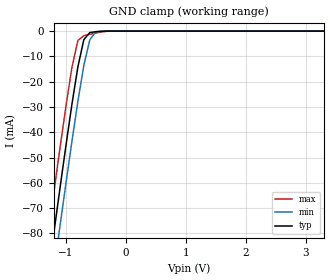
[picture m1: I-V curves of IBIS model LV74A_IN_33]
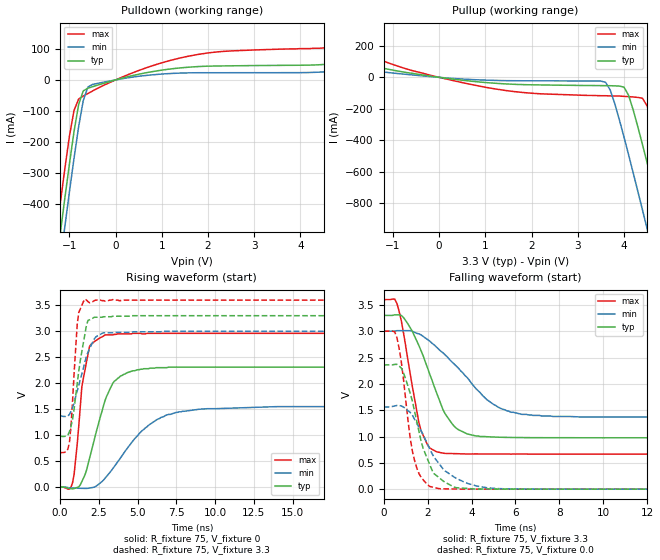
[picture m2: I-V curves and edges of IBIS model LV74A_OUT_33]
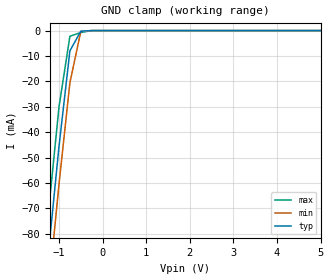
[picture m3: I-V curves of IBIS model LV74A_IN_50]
| TEXAS INSTRUMENTS INCORPORATED
| Standard Linear and Logic Group
| IBIS Model of SN74LV74A
| DUAL POSITIVE-EDGE-TRIGGERED D-TYPE FLIP-FLOPS
| SOIC 14-pin (D), SOP 14-pin (NS), SSOP 14-pin (DB), TSSOP 14-pin (PW)
| and TVSOP 14-pin (DGV) Package
[IBIS Ver]   3.2
[Comment Char]  |_char
[File Name]   sn74lv74a.ibs
[File Rev]   2.1 H_die
[Date]   Nov, 10 2004
[Source]   Data created from HSPICE simulations at TI-SLL.
[Notes]   The following is an IBIS list for the LV74A.
   - FILE REV HISTORY
   - 2.1 Re-Release IBIS file on 11/22/04
   - Power clamp data deleted as there is no power-clamp diode
|   Please contact sllibis@ti.com with questions and
|   comments concerning SLL IBIS models.
[Disclaimer] Property of Texas Instruments Incorporated.  Unauthorized
   reproduction and/or distribution is strictly prohibited.
   This product is protected under copyright law.
   Created 2000, (C) Copyright 2000, Texas Instruments Inc.,
   All Rights Reserved.
   UNLESS THERE IS A SIGNED, WRITTEN AGREEMENT TO THE
   CONTRARY, TEXAS INSTRUMENTS () IS PROVIDING THE IBIS
   MODELS  AND WITHOUT ANY WARRANTY, EXPRESSED OR
   IMPLIED.  TI assumes no liability for:
   1) the accuracy of the IBIS models provided to your
   company;
   2) the proper functioning of these IBIS Models in your
   design or for any resulting applications; or
   3) infringement of patents, copyrights or intellectual
   property rights resulting from your use of these IBIS
   models.
   TI provides IBIS Models as a service to our customers.
   You and your company shall not distribute, sell or give
   these models to anyone else without prior written
   permission from TI.
   TI reserves the right to make changes to our products or
   to discontinue any semiconductor product or service
   without notice, and advises our customers to obtain the
   latest version of relevant information to verify, before
   placing orders, that the information being relied on is
   current.
   Please be aware that your receipt and use of the IBIS
   information provided shall serve as acceptance of these
   terms and conditions.  If you do not accept these terms,
   you should return or destroy the IBIS models and any
   other accompanying information immediately.
|   Component LV74A_D
[Component]   LV74A_D
[Manufacturer]  Texas Instruments, Inc.
[Package]
|   typ   min   max
R_pkg   0.031   0.028   0.034
L_pkg   3.109nH   2.462nH   3.889nH
C_pkg   0.473pF   0.363pF   0.628pF
[Pin]   signal_name   model_name   R_pin   L_pin   C_pin
1   1CLR_NOT   LV74A_IN   0.033   3.854nH   0.622pF
2   1D   LV74A_IN   0.032   3.188nH   0.473pF
3   1CLK   LV74A_IN   0.028   2.462nH   0.377pF
4   1PRE_NOT   LV74A_IN   0.031   2.596nH   0.363pF
5   1Q   LV74A_OUT   0.028   2.521nH   0.372pF
6   1Q_NOT   LV74A_OUT   0.034   3.250nH   0.476pF
7   GND   GND   0.034   3.889nH   0.628pF
8   2Q_NOT   LV74A_OUT   0.034   3.889nH   0.628pF
9   2Q   LV74A_OUT   0.034   3.250nH   0.476pF
10   2PRE_NOT   LV74A_IN   0.028   2.521nH   0.372pF
11   2CLK   LV74A_IN   0.031   2.596nH   0.364pF
12   2D   LV74A_IN   0.028   2.462nH   0.377pF
13   2CLR_NOT   LV74A_IN   0.032   3.188nH   0.473pF
14   VCC   POWER   0.033   3.854nH   0.622pF
|   Component LV74A_NS
[Component]   LV74A_NS
[Manufacturer]  Texas Instruments, Inc.
[Package]
|   typ   min   max
R_pkg   0.045   0.039   0.054
L_pkg   3.796nH   2.561nH   4.952nH
C_pkg   0.528pF   0.288pF   0.710pF
[Pin]   signal_name   model_name   R_pin   L_pin   C_pin
1   1CLR_NOT   LV74A_IN   0.047   4.867nH   0.706pF
2   1D   LV74A_IN   0.051   4.083nH   0.592pF
3   1CLK   LV74A_IN   0.041   2.915nH   0.376pF
4   1PRE_NOT   LV74A_IN   0.039   2.561nH   0.288pF
5   1Q   LV74A_OUT   0.041   3.101nH   0.430pF
6   1Q_NOT   LV74A_OUT   0.047   4.047nH   0.589pF
7   GND   GND   0.051   4.909nH   0.700pF
8   2Q_NOT   LV74A_OUT   0.045   4.784nH   0.694pF
9   2Q   LV74A_OUT   0.054   4.176nH   0.597pF
10   2PRE_NOT   LV74A_IN   0.039   3.287nH   0.449pF
11   2CLK   LV74A_IN   0.039   2.586nH   0.294pF
12   2D   LV74A_IN   0.040   2.802nH   0.371pF
13   2CLR_NOT   LV74A_IN   0.049   4.080nH   0.593pF
14   VCC   POWER   0.052   4.952nH   0.710pF
|   Component LV74A_DB
[Component]   LV74A_DB
[Manufacturer]  Texas Instruments, Inc.
[Package]
|   typ   min   max
R_pkg   0.044   0.041   0.046
L_pkg   3.551nH   3.258nH   3.927nH
C_pkg   0.402pF   0.360pF   0.421pF
[Pin]   signal_name   model_name   R_pin   L_pin   C_pin
1   1CLR_NOT   LV74A_IN   0.046   3.927nH   0.408pF
2   1D   LV74A_IN   0.044   3.587nH   0.421pF
3   1CLK   LV74A_IN   0.041   3.289nH   0.398pF
4   1PRE_NOT   LV74A_IN   0.042   3.258nH   0.360pF
5   1Q   LV74A_OUT   0.041   3.286nH   0.403pF
6   1Q_NOT   LV74A_OUT   0.044   3.586nH   0.421pF
7   GND   GND   0.046   3.927nH   0.408pF
8   2Q_NOT   LV74A_OUT   0.046   3.927nH   0.408pF
9   2Q   LV74A_OUT   0.044   3.586nH   0.421pF
10   2PRE_NOT   LV74A_IN   0.041   3.286nH   0.403pF
11   2CLK   LV74A_IN   0.043   3.258nH   0.360pF
12   2D   LV74A_IN   0.041   3.289nH   0.398pF
13   2CLR_NOT   LV74A_IN   0.044   3.587nH   0.421pF
14   VCC   POWER   0.046   3.927nH   0.408pF
|   Component LV74A_PW
[Component]   LV74A_PW
[Manufacturer]  Texas Instruments, Inc.
[Package]
|   typ   min   max
R_pkg   0.032   0.029   0.035
L_pkg   2.378nH   2.170nH   2.680nH
C_pkg   0.314pF   0.270pF   0.335pF
[Pin]   signal_name   model_name   R_pin   L_pin   C_pin
1   1CLR_NOT   LV74A_IN   0.033   2.618nH   0.330pF
2   1D   LV74A_IN   0.031   2.313nH   0.317pF
3   1CLK   LV74A_IN   0.030   2.310nH   0.314pF
4   1PRE_NOT   LV74A_IN   0.031   2.173nH   0.272pF
5   1Q   LV74A_OUT   0.030   2.204nH   0.309pF
6   1Q_NOT   LV74A_OUT   0.032   2.315nH   0.317pF
7   GND   GND   0.035   2.680nH   0.335pF
8   2Q_NOT   LV74A_OUT   0.033   2.640nH   0.333pF
9   2Q   LV74A_OUT   0.034   2.347nH   0.319pF
10   2PRE_NOT   LV74A_IN   0.029   2.277nH   0.313pF
11   2CLK   LV74A_IN   0.031   2.170nH   0.270pF
12   2D   LV74A_IN   0.031   2.244nH   0.311pF
13   2CLR_NOT   LV74A_IN   0.033   2.343nH   0.321pF
14   VCC   POWER   0.035   2.657nH   0.332pF
|   Component LV74A_DGV
[Component]   LV74A_DGV
[Manufacturer]  Texas Instruments, Inc.
[Package]
|   typ   min   max
R_pkg   0.035   0.020   0.045
L_pkg   2.499nH   2.077nH   2.966nH
C_pkg   0.361pF   0.305pF   0.416pF
[Pin]   signal_name   model_name   R_pin   L_pin   C_pin
1   1CLR_NOT   LV74A_IN   0.027   2.717nH   0.373pF
2   1D   LV74A_IN   0.037   2.434nH   0.398pF
3   1CLK   LV74A_IN   0.034   2.200nH   0.316pF
4   1PRE_NOT   LV74A_IN   0.020   2.077nH   0.309pF
5   1Q   LV74A_OUT   0.030   2.147nH   0.305pF
6   1Q_NOT   LV74A_OUT   0.042   2.580nH   0.408pF
7   GND   GND   0.039   2.921nH   0.385pF
8   2Q_NOT   LV74A_OUT   0.033   2.841nH   0.380pF
9   2Q   LV74A_OUT   0.042   2.611nH   0.410pF
10   2PRE_NOT   LV74A_IN   0.038   2.331nH   0.329pF
11   2CLK   LV74A_IN   0.026   2.223nH   0.319pF
12   2D   LV74A_IN   0.034   2.259nH   0.313pF
13   2CLR_NOT   LV74A_IN   0.045   2.681nH   0.416pF
14   VCC   POWER   0.042   2.966nH   0.386pF
[Model Selector]   LV74A_IN
LV74A_IN_33   3.3-V Vcc Input Model
LV74A_IN_50   5.0-V Vcc Input Model
[Model Selector]   LV74A_OUT
LV74A_OUT_33   3.3-V Vcc Output Model
LV74A_OUT_50   5.0-V Vcc Output Model
| Models and submodels in the file (4): LV74A_IN_33 (Input), LV74A_OUT_33 (Output), LV74A_IN_50 (Input), LV74A_OUT_50 (Output)
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|   Model LV74A_IN_33
[Model]   LV74A_IN_33
Model_type  Input
Polarity   Inverting
Vinl = 0.99
Vinh = 2.31
| variable   typ   min   max
C_comp   1.24pf   0.94pf   1.54pf
[Temperature Range]   25   85   -40
[Voltage Range]   3.3   3.0   3.6
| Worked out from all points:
|   GND clamp passes 1 mA (typ) near -0.61 V on its own axis
[GND Clamp]
|   Voltage   I(typ)   I(min)   I(max)
-3.3V     -460mA     -475mA     -445mA
-1.3V     -97.5mA    -113mA     -81.5mA
-1.2V     -79.9mA    -95mA      -63.9mA
-1.1V     -62.6mA    -77.6mA    -46.7mA
-1V       -45.6mA    -60.5mA    -30mA
-900mV    -29.2mA    -43.9mA    -14.6mA
-800mV    -14.3mA    -28mA      -3.81mA
-700mV    -3.42mA    -13.6mA    -1.78mA
-600mV    -581uA     -3.4mA     -1.25mA
-500mV    -233uA     -353uA     -759uA
-400mV    -58.1uA    -21.9uA    -324uA
3.3V      1.9nA      2.34nA     1.69nA
|   Model LV74A_OUT_33
[Model]   LV74A_OUT_33
Model_type  Output
Polarity   Non-Inverting
Vmeas = 1.65v
Cref = 15pf
| variable   typ   min   max
C_comp   4.62pf   3.47pf   5.77pf
[Temperature Range]   25   85   -40
[Voltage Range]   3.3   3.0   3.6
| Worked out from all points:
|   slope of the pulldown table from 0 to 0.495 V, typ, clamps not added: 27.3 ohm
|   slope of the pullup table from 0 to 0.495 V, typ, clamps not added: 27.2 ohm
|   rising waveform, R_fixture 75, V_fixture 0: 20-80 % time 1.34ns typ, 2.67ns min, 654ps max; typ from 0.002 V to 2.31 V
|   falling waveform, R_fixture 75, V_fixture 3.3: 20-80 % time 1.3ns typ, 2.25ns min, 730ps max; typ from 3.3 V to 0.976 V
|   rising waveform, R_fixture 75, V_fixture 3.3: 20-80 % time 664ps typ, 943ps min, 358ps max; typ from 0.976 V to 3.3 V
|   falling waveform, R_fixture 75, V_fixture 0.0: 20-80 % time 936ps typ, 1.4ns min, 568ps max; typ from 2.36 V to 0 V
[Pulldown]
|   Voltage   I(typ)   I(min)   I(max)
-3.3V     -3.04A     -3.13A     -2.95A
-1.3V     -615mA     -707mA     -518mA
-1.2V     -498mA     -591mA     -401mA
-1.1V     -383mA     -475mA     -288mA
-900mV    -167mA     -253mA     -98.6mA
-800mV    -79.1mA    -151mA     -61.7mA
-700mV    -35.5mA    -66.4mA    -51.9mA
-600mV    -26.8mA    -23.2mA    -43.9mA
-500mV    -22mA      -14.7mA    -35.8mA
1.6V      41.2mA     22.8mA     77.1mA
4.7V      52.1mA     27.5mA     106mA
6.6V      86.8mA     47.3mA     166mA
[Pullup]
|   Voltage   I(typ)   I(min)   I(max)
-3.3V     166mA      91.1mA     311mA
600mV     -21.6mA    -12.3mA    -39.7mA
3.6V      -52.9mA    -31.5mA    -117mA
3.8V      -54.2mA    -168mA     -119mA
4V        -62.6mA    -381mA     -121mA
4.1V      -115mA     -494mA     -123mA
4.4V      -429mA     -845mA     -133mA
4.5V      -544mA     -964mA     -182mA
4.8V      -899mA     -1.32A     -505mA
4.9V      -1.02A     -1.44A     -622mA
5.2V      -1.38A     -1.81A     -981mA
6.6V      -3.09A     -3.52A     -2.69A
[Ramp]
| variable   typ   min   max
dV/dt_r   1.40E+00/1.33E-09   9.37E-01/2.69E-09   1.78E+00/5.76E-10
dV/dt_f   1.41E+00/1.33E-09   9.88E-01/2.26E-09   1.77E+00/7.47E-10
R_load = 75
[Rising Waveform]
R_fixture = 75
V_fixture = 0
|   Time   V(typ)   V(min)   V(max)
0s        1.61mV     1.45mV     1.35mV
800ps     -32.5mV    -18.2mV    84mV
1.1ns     -5.95mV    -20.8mV    827mV
1.4ns     107mV      -23.1mV    1.93V
1.9ns     558mV      -17.4mV    2.71V
2.9ns     1.67V      172mV      2.93V
4.3ns     2.2V       735mV      2.95V
5.7ns     2.28V      1.19V      2.96V
7.5ns     2.31V      1.44V      2.96V
25ns      2.31V      1.55V      2.96V
[Falling Waveform]
R_fixture = 75
V_fixture = 3.3
V_fixture_min = 3.0
V_fixture_max = 3.6
|   Time   V(typ)   V(min)   V(max)
0s        3.3V       3V         3.6V
600ps     3.31V      3.01V      3.53V
1.1ns     3.14V      3.01V      2.46V
1.7ns     2.63V      2.93V      1.11V
2.4ns     1.84V      2.7V       711mV
2.8ns     1.43V      2.55V      679mV
3.4ns     1.13V      2.3V       673mV
4.7ns     996mV      1.7V       667mV
6.3ns     980mV      1.42V      667mV
25ns      976mV      1.37V      666mV
[Rising Waveform]
R_fixture = 75
V_fixture = 3.3
V_fixture_min = 3.0
V_fixture_max = 3.6
|   Time   V(typ)   V(min)   V(max)
0s        976mV      1.37V      666mV
400ps     981mV      1.36V      688mV
600ps     1.07V      1.4V       858mV
700ps     1.17V      1.46V      1.17V
1.1ns     1.99V      1.85V      3.13V
1.2ns     2.23V      1.96V      3.36V
1.6ns     2.95V      2.41V      3.62V
1.8ns     3.21V      2.6V       3.57V
2.8ns     3.28V      2.97V      3.59V
25ns      3.3V       3V         3.6V
[Falling Waveform]
R_fixture = 75
V_fixture = 0.0
|   Time   V(typ)   V(min)   V(max)
0s        2.36V      1.56V      3V
600ps     2.37V      1.59V      2.88V
800ps     2.3V       1.58V      2.42V
1.3ns     1.68V      1.41V      732mV
1.6ns     1.11V      1.18V      302mV
2.1ns     463mV      763mV      51.3mV
2.3ns     292mV      604mV      31.5mV
3.2ns     40.7mV     232mV      3.33mV
4.8ns     4.38mV     22.6mV     737uV
25ns      10.7uV     562nV      13.8uV
|   Model LV74A_IN_50
[Model]   LV74A_IN_50
Model_type  Input
Polarity   Inverting
Vinl = 1.5
Vinh = 3.5
| variable   typ   min   max
C_comp   1.24pf   0.94pf   1.54pf
[Temperature Range]   25   85   -40
[Voltage Range]   5.0   4.5   5.5
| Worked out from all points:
|   GND clamp passes 1 mA (typ) near -0.52 V on its own axis
[GND Clamp]
|   Voltage   I(typ)   I(min)   I(max)
-5V       -773mA     -786mA     -758mA
-1.5V     -133mA     -148mA     -117mA
-1.25V    -88.7mA    -104mA     -72.7mA
-1V       -45.6mA    -60.5mA    -30mA
-750mV    -7.99mA    -20.5mA    -2.23mA
-500mV    -233uA     -353uA     -759uA
-250mV    -2.63nA    -182nA     -26.9uA
5V        2.9nA      3.64nA     2.54nA
